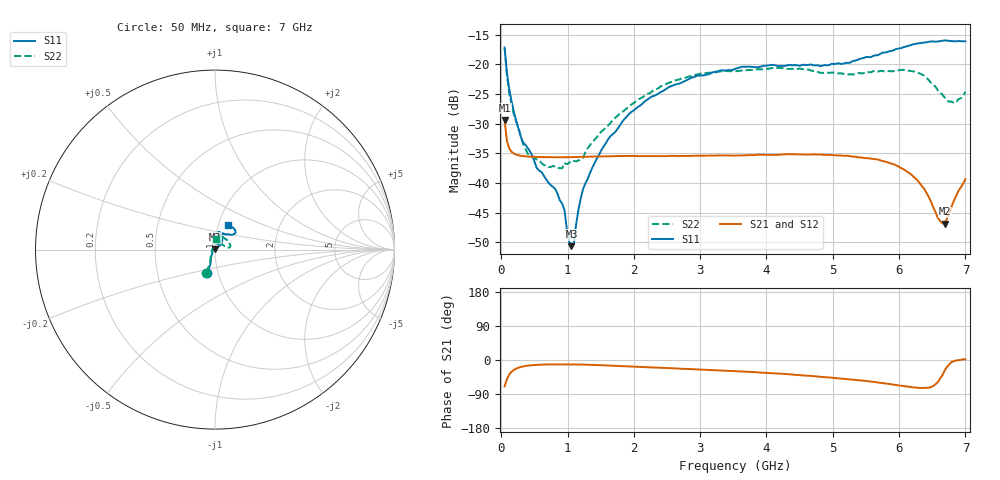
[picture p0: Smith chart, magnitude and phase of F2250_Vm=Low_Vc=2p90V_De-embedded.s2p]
! Integrated Device Technology
! Corporate Headquarters
! 6024 Silver Creek Valley Road
! San Jose, CA 95138  USA
! Phone:  1-408-284-8200
! Toll Free:  1-800-223-1366
! Webpage:  http://www.idt.com/
! Timing and RF Division
! 515 Groton Road, Suite 102
! Westford, MA 01886-6024
! Device:  F2250
! Description: Voltage Variable RF Attenuator
! Frequency:  50.0 -  6000.00 MHz
! Package:  3x3 mm Thin QFN Plastic Package: 16 pin
! Ports:  2 RF, 3 DC
!  Pin  1  = GND
!  Pin  2  = NC
!  Pin  3  = RF1  = Port 1
!  Pin  4  = NC
!  Pin  5  = GND
!  Pin  6  = GND
!  Pin  7  = GND
!  Pin  8  = GND
!  Pin  9  = NC
!  Pin 10  = RF2  = Port 2
!  Pin 11  = NC
!  Pin 12  = GND
!  Pin 13  = GND
!  Pin 14  = VCNTRL
!  Pin 15  = VDD
!  Pin 16  = VMODE
! Vcntrl:  2.900 Volts
! Vmode:  +0.000 Volts
! Vdd:  +3.30  Volts
! Current:  1.175 mA
! Data:  The device was measured on a the F2250 evaluation board which has
!  individual transmission lines to the RF pins.  Data was collected
!  using a calibrated network analyzer.  The evaluation board was
!  de-embedded using a TRL calibration technique.
!  The reference plane is the edge of the package pin.
! Misc:  SN 10
!  Action Tracker AT0258
! Date Measured:  2014-11-26
! Date:  2015-10-15  MJV
! Note:
!  Integrated Device Technology supplies this data as a sample of measured
!  data at the package pin for this product.  Your particular data for this
!  product may vary.
!  Data was taken at 25 degrees C.
!  Integrated Device Technology reserves the right to change this data at anytime.
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# GHz S dB R 50
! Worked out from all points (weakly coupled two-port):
!   201 points, 50 MHz to 7 GHz, reference 50 ohm
!   highest |S21| = -29.41 dB at 50 MHz (marker M1); lowest = -46.9 dB at 6.687 GHz (marker M2)
!   lowest |S11| = -50.7 dB at 1.058 GHz (marker M3), VSWR 1.01, Z = 49.8 + j0.243 ohm
!   |S11| at or under -10 dB: start of sweep to end of sweep
!   |S22| runs from -37.5 to -17.3 dB; largest |S21 - S12| = 6.4e-05
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0.05  -17.18 -108.6  -29.41 -69.8  -29.41 -69.8  -17.28 -111.0
0.08475  -21.45 -107.5  -32.92 -50.4  -32.92 -50.4  -21.75 -110.2
0.15425  -26.23 -116.6  -34.75 -31.1  -34.76 -31.1  -26.81 -122.4
0.29325  -32.21 -127.9  -35.43 -18.5  -35.43 -18.5  -32.09 -137.4
0.3975  -34.09 -141.8  -35.56 -15.0  -35.56 -15.0  -35.04 -160.4
0.91875  -43.50 157.9  -35.68 -11.5  -35.68 -11.5  -37.54 133.5
0.9535  -44.61 170.1  -35.68 -11.5  -35.68 -11.5  -36.64 131.2
1.023  -49.91 143.4  -35.67 -11.6  -35.67 -11.6  -36.63 115.9
1.05775  -50.67 123.5  -35.67 -11.6  -35.67 -11.6  -36.26 110.7
1.0925  -50.44 89.8  -35.66 -11.7  -35.66 -11.7  -36.31 106.4
1.162  -44.68 56.8  -35.64 -11.9  -35.64 -11.9  -36.21 95.6
1.2315  -41.11 44.1  -35.61 -12.1  -35.61 -12.1  -35.79 85.8
1.6485  -32.11 41.9  -35.52 -14.7  -35.52 -14.6  -29.87 64.5
1.96125  -28.05 42.2  -35.46 -17.2  -35.46 -17.2  -26.80 56.8
2.37825  -24.87 47.3  -35.48 -20.3  -35.48 -20.3  -23.99 56.7
3.525  -20.79 72.5  -35.40 -29.6  -35.40 -29.6  -21.19 74.7
4.7065  -20.17 72.3  -35.19 -42.6  -35.19 -42.6  -21.14 72.2
5.85325  -17.82 40.5  -36.63 -63.4  -36.63 -63.5  -21.14 23.1
6.27025  -16.51 40.0  -39.50 -72.8  -39.51 -72.9  -21.37 9.7
6.68725  -15.99 48.7  -46.89 -27.9  -46.89 -27.4  -25.63 28.7
6.861  -16.14 55.1  -42.19 -1.3  -42.16 -1.4  -26.46 57.9
7  -16.13 63.2  -39.37 1.9  -39.32 1.7  -24.63 83.0
